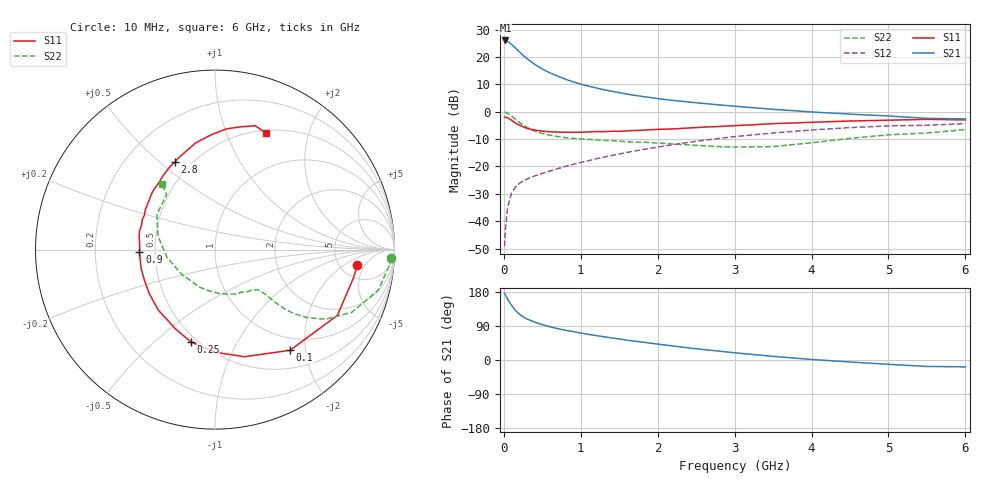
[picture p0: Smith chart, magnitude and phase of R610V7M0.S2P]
! SIEMENS Small Signal Semiconductors
! BFR193
! Si NPN RF Bipolar Junction Transistor in SOT23
! VCE = 10 V  IC = 7 mA
! Common Emitter S-Parameters:  May  1996
# GHz  S  MA  R  50
!  f  S11  S21  S12  S22
! GHz  MAG  ANG  MAG  ANG  MAG  ANG  MAG  ANG
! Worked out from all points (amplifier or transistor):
!   36 points, 10 MHz to 6 GHz, reference 50 ohm
!   highest |S21| = 26.0 dB at 20 MHz (marker M1)
!   |S21| within 3 dB of that: start of sweep to 159.9 MHz
!   unconditionally stable (mu >= 1): 847.8 MHz to 2.05 GHz
!   at 250 MHz: K = 0.51, MSG = 22.9 dB, |S12| = -25.3 dB
!   at 1.4 GHz: K = 1.05, MAG = 10.4 dB, |S12| = -16.0 dB
!   at 6 GHz: K = 0.94, MSG = 0.9 dB, |S12| = -4.4 dB
!   S11 on the Smith chart (normalised r, x): 10 MHz: 7.33, -3.36; 100 MHz: 0.78, -1.72; 250 MHz: 0.46, -0.66; 900 MHz: 0.41, -0.01; 2.8 GHz: 0.41, +0.56; 6 GHz: 0.53, +1.39
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0.01  0.7979 -6.0  19.93 176.0  0.0035 81.9  0.9825 -2.8
0.02  0.7873 -11.6  20.01 171.7  0.0073 79.2  0.9723 -5.7
0.05  0.7743 -28.2  19.29 160.5  0.0182 75.4  0.9372 -14.0
0.1  0.6997 -53.3  16.99 144.3  0.0327 65.2  0.8375 -24.7
0.15  0.6191 -74.6  14.63 130.7  0.0421 58.5  0.728 -32.2
0.2  0.5704 -91.0  12.45 121.5  0.0488 55.0  0.6394 -36.4
0.25  0.5309 -104.8  10.67 114.0  0.0546 52.5  0.5703 -38.9
0.3  0.4949 -116.0  9.336 108.2  0.0587 52.2  0.5164 -40.3
0.4  0.4618 -133.3  7.371 100.0  0.0669 52.2  0.443 -41.3
0.5  0.441 -145.8  5.996 93.2  0.0746 53.3  0.4 -41.4
0.6  0.429 -156.3  5.113 87.7  0.0826 54.5  0.3726 -41.6
0.7  0.4248 -165.2  4.46 82.7  0.0912 56.4  0.3516 -42.1
0.9  0.4209 -178.0  3.512 74.8  0.1092 58.4  0.3247 -43.4
1.1  0.4277 170.9  2.937 67.7  0.1274 59.4  0.3128 -46.4
1.3  0.4316 161.4  2.521 61.4  0.1481 59.9  0.3004 -49.7
1.6  0.4478 150.0  2.098 52.4  0.18 59.6  0.2833 -56.6
2.2  0.4848 130.8  1.605 36.9  0.2505 55.9  0.2575 -74.7
2.8  0.5376 114.6  1.333 23.3  0.325 49.4  0.2306 -101.2
3.5  0.6044 100.3  1.105 9.6  0.4084 39.2  0.2306 -142.9
4.5  0.6755 84.6  0.903 -5.3  0.5132 24.1  0.3256 167.0
5.5  0.7254 72.1  0.756 -17.0  0.5664 7.8  0.4087 131.2
6  0.7089 66.2  0.738 -18.1  0.6053 3.1  0.4716 129.1
